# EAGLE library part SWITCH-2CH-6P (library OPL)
6P-2CH-2.54-L9.0*W3.5*H3.2+2.0MM:311010004;6P-2CH-2.54-L9.0*W3.5*H3.2-90D:311030004;6P-2CH-2.54-SMD-L7.0*W3.5*H1.5MM:311030005
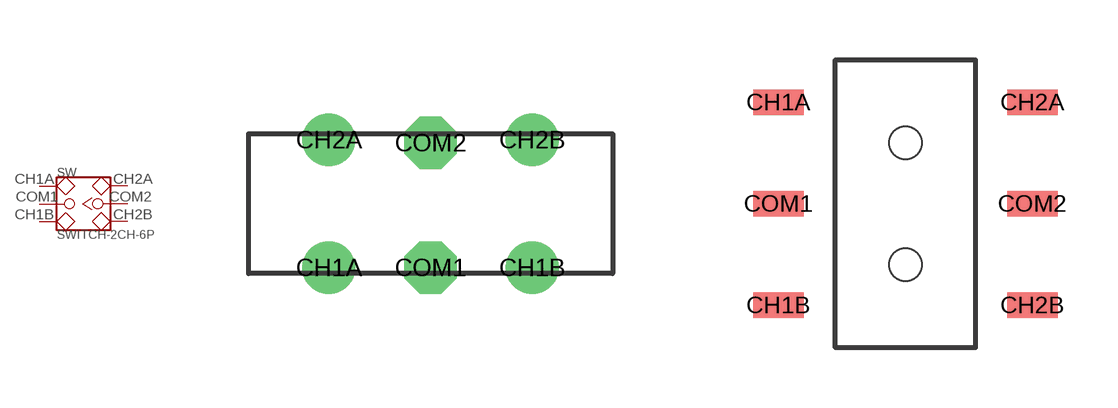
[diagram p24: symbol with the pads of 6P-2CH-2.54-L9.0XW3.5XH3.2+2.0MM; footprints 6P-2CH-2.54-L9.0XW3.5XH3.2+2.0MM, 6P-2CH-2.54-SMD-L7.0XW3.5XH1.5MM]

Designator prefix SW

## SWITCH-2CH-6P-MS-22D18  [6P-2CH-2.54-L9.0XW3.5XH3.2+2.0MM]
CH1A  CH1A
CH1B  CH1B
CH2A  CH2A
CH2B  CH2B
COM1  COM1
COM2  COM2

## SWITCH-2CH-6P-311030005  [6P-2CH-2.54-SMD-L7.0XW3.5XH1.5MM]
Pads as for 6P-2CH-2.54-L9.0XW3.5XH3.2+2.0MM

## SWITCH-2CH-6P-90D  [6P-2CH-2.54-L9.0XW3.5XH3.2-90D]
Pads as for 6P-2CH-2.54-L9.0XW3.5XH3.2+2.0MM

## Footprint 6P-2CH-2.54-L9.0XW3.5XH3.2+2.0MM (pad centres in mm)
drill 0.813 pad 1.27: CH1A -2.54,-1.6; CH1B 2.54,-1.6; CH2A -2.54,1.6; CH2B 2.54,1.6
drill 0.813 pad 1.27 octagon: COM1 0,-1.6; COM2 0,1.524

## Footprint 6P-2CH-2.54-SMD-L7.0XW3.5XH1.5MM (pad centres in mm)
smd 1.27 x 0.635: CH1A -3.175,2.54; CH1B -3.175,-2.54; CH2A 3.175,2.54; CH2B 3.175,-2.54; COM1 -3.175,0; COM2 3.175,0
hole 0.813 at 0,1.524
hole 0.813 at 0,-1.524

## Footprint 6P-2CH-2.54-L9.0XW3.5XH3.2-90D (pad centres in mm)
drill 0.813 pad 1.27: CH1A -2.54,-1.65; CH1B 2.54,-1.65; CH2A -2.54,1.65; CH2B 2.54,1.65
drill 0.813 pad 1.27 octagon: COM1 0,-1.65; COM2 0,1.65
